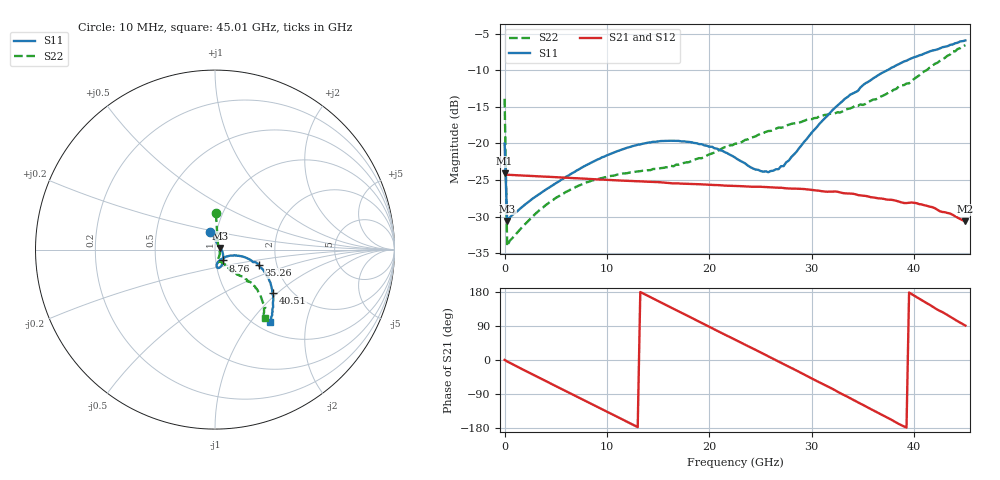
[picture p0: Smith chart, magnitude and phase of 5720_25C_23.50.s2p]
! Device:  ADRF5720
! Description: 0.5dB LSB GaAs MMIC 6-bit Digital Attenuator
! Frequency:  0.000009 -  40 GHz
! Ports:
!	RF1	= Port 1
!	RF2	= Port 2
! Vdd:  3.3 Volt
! Vss:  -3.3 Volt
! Control:  0/3.3 Volt
! State:  23.50 dB attenuation
! Data:  The device was measured using G-S-G Probes on a matrix board.
!  Data was collected using an calibrated 4 port network analyzer.
!  The reference plane for this measurement is at the launchers.
! Note:  Analog Devices supplies this data as a sample of measured data
!  for this product.  Your particular data for this product may vary.
!  Data was taken at 25 degrees C.
!  Analog Devices reserves the right to change this data at anytime.
# GHZ S DB R 45.0
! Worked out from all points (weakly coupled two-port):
!   181 points, 10 MHz to 45.01 GHz, reference 45 ohm
!   highest |S21| = -24.09 dB at 10 MHz (marker M1); lowest = -30.7 dB at 45.01 GHz (marker M2)
!   lowest |S11| = -30.6 dB at 260 MHz (marker M3), VSWR 1.06, Z = 47.6 + j0.863 ohm
!   |S11| at or under -10 dB: start of sweep to 37.34 GHz
!   |S22| runs from -34.1 to -6.6 dB; largest |S21 - S12| = 0.00015
!   S11 on the Smith chart (normalised r, x): 10 MHz: 0.93, +0.18; 8.76 GHz: 1.09, -0.13; 35.26 GHz: 1.61, -0.30; 40.51 GHz: 1.62, -0.92; 45.01 GHz: 1.15, -1.25
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0.01  -20.02 104.9  -24.09 0.1  -24.09 0.1  -13.88 88.7
0.26  -30.62 17.9  -24.28 -3.8  -24.29 -3.8  -34.06 24.6
0.51  -30.13 9.5  -24.30 -7.3  -24.31 -7.3  -33.32 10.5
3.51  -26.82 -21.1  -24.51 -48.5  -24.51 -48.5  -29.03 -40.9
5.01  -25.44 -32.5  -24.61 -68.9  -24.62 -68.8  -27.45 -55.1
7.76  -23.14 -48.1  -24.82 -106.1  -24.81 -106.1  -25.47 -69.8
8.760001  -22.43 -52.9  -24.89 -119.6  -24.89 -119.6  -25.00 -72.7
12.01  -20.57 -65.8  -25.11 -163.6  -25.11 -163.5  -24.06 -76.8
15.26  -19.67 -76.0  -25.32 151.9  -25.32 151.9  -23.38 -73.2
19.26  -20.10 -84.1  -25.60 97.7  -25.60 97.7  -22.02 -62.7
22.76  -22.17 -81.4  -25.83 50.3  -25.84 50.3  -20.02 -55.9
25.26  -23.86 -60.6  -25.95 16.4  -25.95 16.4  -18.59 -54.4
26.76  -23.52 -41.5  -26.06 -3.9  -26.05 -3.8  -17.82 -53.0
27.76  -22.34 -29.3  -26.16 -17.6  -26.16 -17.5  -17.44 -53.1
30.26  -18.12 -15.2  -26.40 -52.1  -26.40 -52.1  -16.52 -52.5
32.26  -15.13 -14.5  -26.57 -79.5  -26.57 -79.5  -15.89 -50.8
35.26  -11.75 -19.4  -27.18 -122.2  -27.18 -122.2  -14.58 -47.2
37.76  -9.66 -27.4  -27.71 -157.3  -27.70 -157.2  -12.93 -43.6
40.51  -7.94 -36.7  -28.31 161.7  -28.32 161.7  -10.67 -43.0
42.26  -7.13 -42.8  -29.06 133.1  -29.06 133.0  -8.97 -45.0
43.76  -6.45 -48.1  -29.76 110.1  -29.77 110.1  -7.37 -49.1
45.01  -5.90 -53.0  -30.68 90.9  -30.68 91.0  -6.55 -53.8
